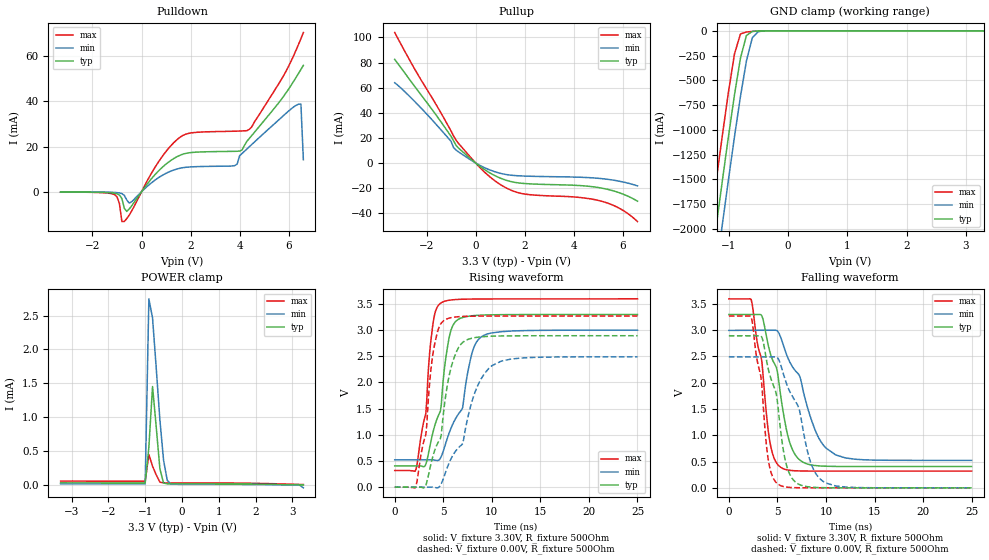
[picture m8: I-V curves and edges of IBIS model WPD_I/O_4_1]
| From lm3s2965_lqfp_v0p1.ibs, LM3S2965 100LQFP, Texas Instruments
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[Model]   WPD_I/O_4_1
Model_type   I/O
Vinl = 1.26
Vinh = 2.04
Vmeas = 1.65
| variable   typ   min   max
C_comp   9.739pF   9.739pF   9.739pF
[Model Spec]
Vinh+   1.91   1.78   2.04
Vinh-   1.90   1.76   2.03
Vinl+   1.40   1.27   1.54
Vinl-   1.39   1.26   1.53
| variable   typ   min   max
[Temperature Range]  25   85   -40
[Voltage Range]   3.3V   3.0V   3.6V
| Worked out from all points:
|   slope of the pulldown table from 0 to 0.495 V, typ, clamps not added: 71.6 ohm
|   slope of the pullup table from 0 to 0.495 V, typ, clamps not added: 71.6 ohm
|   GND clamp passes 1 mA (typ) near -0.48 V on its own axis
|   POWER clamp passes 1 mA (typ) near -0.72 V on its own axis
|   falling waveform, V_fixture 3.30V, R_fixture 500Ohm: 20-80 % time 2.03ns typ, 3.06ns min, 1.36ns max; typ from 3.3 V to 0.405 V
|   rising waveform, V_fixture 3.30V, R_fixture 500Ohm: 20-80 % time 1.61ns typ, 2.31ns min, 1.11ns max; typ from 0.405 V to 3.3 V
|   falling waveform, V_fixture 0.00V, R_fixture 500Ohm: 20-80 % time 1.75ns typ, 2.48ns min, 1.21ns max; typ from 2.89 V to 0 V
|   rising waveform, V_fixture 0.00V, R_fixture 500Ohm: 20-80 % time 1.94ns typ, 2.99ns min, 1.26ns max; typ from 0 V to 2.89 V
[Pulldown]
|  Voltage   I(typ)   I(min)   I(max)
-3.3V     -128.2uA   -72.79uA   -182.2uA
-1.1V     -636.2uA   -293.6uA   -1.283mA
-800mV    -2.996mA   -834.9uA   -13.19mA
-700mV    -7.354mA   -1.607mA   -13.15mA
-500mV    -7.623mA   -4.999mA   -10.32mA
700mV     9.301mA    6.299mA    13.36mA
1.6V      16.31mA    10.5mA     24.39mA
3.8V      17.93mA    11.6mA     26.84mA
4.4V      23.69mA    19.99mA    27.69mA
6.4V      52.4mA     38.79mA    65.21mA
6.5V      54.19mA    38.86mA    67.83mA
6.6V      55.99mA    14.2mA     70.53mA
[Pullup]
|  Voltage   I(typ)   I(min)   I(max)
-3.3V     82.55mA    63.93mA    103.9mA
-1.8V     43.23mA    34.85mA    52.65mA
-1V       21.12mA    17.2mA     25.41mA
-900mV    17.75mA    12.24mA    21.49mA
-800mV    14.04mA    10.31mA    18.31mA
100mV     -1.569mA   -1.126mA   -2.147mA
700mV     -9.236mA   -6.432mA   -12.93mA
1.3V      -14.09mA   -9.375mA   -20.39mA
1.9V      -16.21mA   -10.36mA   -24.42mA
5.2V      -20.25mA   -12.6mA    -30.84mA
5.9V      -24.02mA   -14.69mA   -36.54mA
6.6V      -30.45mA   -18.28mA   -46.68mA
[GND Clamp]
|  Voltage   I(typ)   I(min)   I(max)
-3.3V     -11.72A    -12.12A    -11.3A
-1.4V     -2.845A    -3.285A    -2.387A
-1.3V     -2.39A     -2.831A    -1.93A
-1.2V     -1.938A    -2.38A     -1.478A
-1.1V     -1.494A    -1.934A    -1.036A
-1V       -1.059A    -1.496A    -610.6mA
-900mV    -645mA     -1.069A    -232.9mA
-800mV    -277.1mA   -664.4mA   -31.59mA
-700mV    -48.56mA   -306.6mA   -12.1mA
-600mV    -5.561mA   -70.2mA    -6.281mA
-500mV    -1.172mA   -7.88mA    -2.176mA
3.3V      16.11uA    11.84uA    29.77uA
[POWER Clamp]
|  Voltage   I(typ)   I(min)   I(max)
-3.3V     31.42uA    17.14uA    57.54uA
-1V       30.25uA    16.5uA     55.43uA
-900mV    557.3uA    2.746mA    449.1uA
-800mV    1.452mA    2.463mA    276.5uA
-700mV    854.2uA    1.726mA    147.8uA
-600mV    235.9uA    958.2uA    41.01uA
-500mV    28.31uA    363.4uA    30.71uA
-400mV    16.41uA    67.09uA    29.83uA
-300mV    16.12uA    11.84uA    29.79uA
3.1V      2.408uA    -920.8nA   9.197uA
3.2V      1.227uA    -3.925uA   7.474uA
3.3V      -104.7pA   -42.65uA   5.692uA
[Ramp]
| variable   typ   min   max
dV/dt_f   1.73/2.03n   1.48/3.06n   1.97/1.36n
dV/dt_r   1.74/1.94n   1.49/2.99n   1.96/1.26n
R_load = 500Ohm
[Falling Waveform]
V_fixture = 3.30V
V_fixture_min = 3.00V
V_fixture_max = 3.60V
R_fixture = 500Ohm
|   Time   V(typ)   V(min)   V(max)
0s        3.297V     2.995V     3.595V
2.3ns     3.297V     2.998V     3.582V
3.4ns     3.272V     2.998V     2.405V
4.2ns     2.605V     2.998V     904.5mV
5.3ns     1.806V     2.883V     396.4mV
6.1ns     972.7mV    2.465V     338.5mV
6.9ns     612mV      2.217V     324.2mV
9.1ns     420.8mV    1.008V     318.9mV
11ns      407.6mV    627mV      318.6mV
25ns      405.4mV    522.4mV    318.5mV
[Rising Waveform]
V_fixture = 3.30V
V_fixture_min = 3.00V
V_fixture_max = 3.60V
R_fixture = 500Ohm
|   Time   V(typ)   V(min)   V(max)
0s        405.4mV    522.4mV    318.5mV
2.2ns     405.4mV    522.4mV    343mV
3.2ns     435.5mV    522.4mV    1.4V
3.6ns     760.2mV    522.3mV    2.571V
4ns       1.092V     521.2mV    3.195V
4.7ns     1.449V     551.8mV    3.511V
5.2ns     2.388V     807.4mV    3.554V
5.9ns     3.051V     1.172V     3.578V
9ns       3.287V     2.881V     3.595V
25ns      3.298V     2.999V     3.597V
[Falling Waveform]
V_fixture = 0.00V
V_fixture_min = 0.00V
V_fixture_max = 0.00V
R_fixture = 500Ohm
|   Time   V(typ)   V(min)   V(max)
0s        2.893V     2.49V      3.27V
2.3ns     2.893V     2.491V     3.256V
3.3ns     2.891V     2.491V     2.119V
4.1ns     2.228V     2.491V     489.2mV
5.1ns     1.475V     2.451V     66.07mV
5.7ns     623.8mV    2.118V     22.43mV
6.4ns     215mV      1.79V      7.113mV
8.5ns     13.49mV    445.2mV    479.7uV
9.7ns     3.634mV    124.5mV    177.5uV
25ns      17.27uV    28.07uV    10.86uV
[Rising Waveform]
V_fixture = 0.00V
V_fixture_min = 0.00V
V_fixture_max = 0.00V
R_fixture = 500Ohm
|   Time   V(typ)   V(min)   V(max)
0s        192.2uV    3.96mV     12.11uV
2.2ns     30.33uV    819.7uV    27.43mV
3.2ns     33.68mV    421.4uV    997.8mV
4ns       634.4mV    -846uV     2.619V
4.7ns     927.2mV    32.83mV    3.106V
5.1ns     1.54V      213mV      3.188V
6.7ns     2.703V     778mV      3.258V
8.4ns     2.86V      1.876V     3.267V
10ns      2.884V     2.319V     3.269V
25ns      2.893V     2.49V      3.269V
